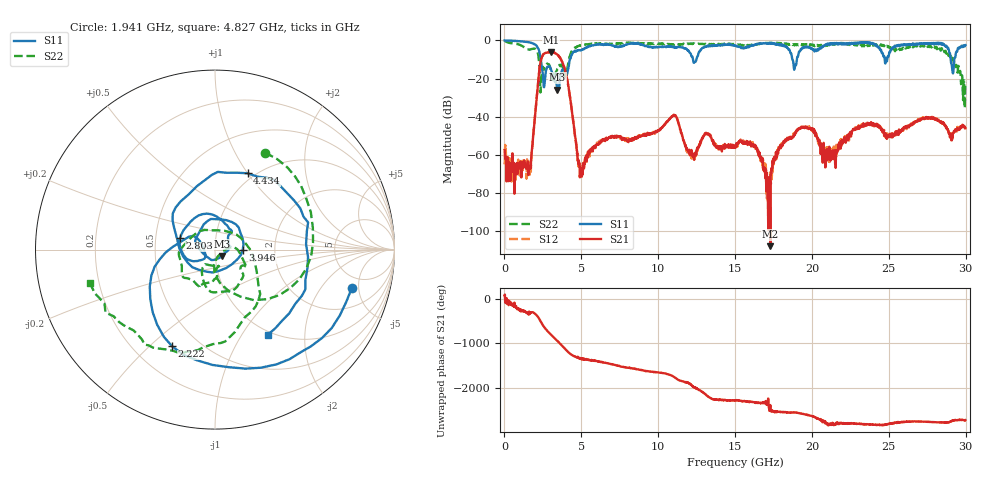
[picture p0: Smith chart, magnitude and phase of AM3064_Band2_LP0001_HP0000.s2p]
# Hz S DB R 50.0
!freq dBS11 angS11 dBS21 angS21 dBS12 angS12 dBS22 angS22
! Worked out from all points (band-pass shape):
!   1600 points, 10 MHz to 29.98 GHz, reference 50 ohm
!   highest |S21| = -6.14 dB at 3.028 GHz (marker M1); lowest = -107.7 dB at 17.29 GHz (marker M2)
!   |S21| within 3 dB of the highest: 2.415 GHz to 3.607 GHz (1.191 GHz wide, 39.6 % of centre)
!   lowest |S11| = -25.7 dB at 3.44 GHz (marker M3), VSWR 1.11, Z = 53.8 - j3.8 ohm
!   |S11| at or under -10 dB: 2.369 GHz to 4.257 GHz (1.888 GHz wide, 57 % of centre); 18.73 GHz to 19.02 GHz (291.7 MHz wide, 1.55 % of centre); 29.03 GHz to 29.26 GHz (229.3 MHz wide, 0.787 % of centre)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
!   |S22| runs from -35.5 to -0.2 dB; largest |S21 - S12| = 0.018
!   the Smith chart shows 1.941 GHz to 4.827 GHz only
!   S11 on the Smith chart (normalised r, x): 1.941 GHz: 3.62, -4.17; 2.222 GHz: 0.36, -0.59; 2.803 GHz: 0.67, +0.09; 3.946 GHz: 1.37, -0.00; 4.434 GHz: 0.92, +1.00; 4.827 GHz: 0.95, -1.31
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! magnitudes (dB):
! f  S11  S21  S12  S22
! 10 MHz  0.0  -57.4  -64.9  -0.2
! 1.566 GHz  -0.9  -66.9  -66.6  -4.7
! 1.941 GHz  -2.0  -43.3  -43.3  -4.3
! 2.222 GHz  -4.6  -19.2  -19.1  -9.0
! 2.803 GHz  -13.7  -6.3  -6.3  -12.3
! 3.028 GHz  -15.1  -6.1  -6.1  -16.6
! 3.44 GHz  -25.7  -7.5  -7.3  -14.9
! 3.946 GHz  -16.2  -15.7  -15.8  -18.1
! 4.434 GHz  -6.7  -39.7  -39.8  -4.9
! 4.827 GHz  -5.1  -63.0  -66.2  -2.8
! 5.015 GHz  -5.0  -68.0  -67.9  -2.6
! 10 GHz  -3.4  -47.2  -47.4  -1.7
! 15 GHz  -2.6  -56.3  -55.4  -1.8
! 17.29 GHz  -1.6  -107.7  -70.0  -1.4
! 18.14 GHz  -3.0  -53.7  -53.0  -1.8
! 19.99 GHz  -4.1  -46.1  -47.0  -2.1
! 21.42 GHz  -1.6  -59.3  -54.8  -1.5
! 23.23 GHz  -1.3  -44.5  -44.2  -2.5
! 25 GHz  -8.0  -50.4  -49.0  -3.1
! 28.56 GHz  -2.1  -43.0  -43.3  -4.9
! 29.18 GHz  -17.2  -48.5  -47.4  -9.3
! 29.98 GHz  -2.4  -46.0  -46.0  -21.7
